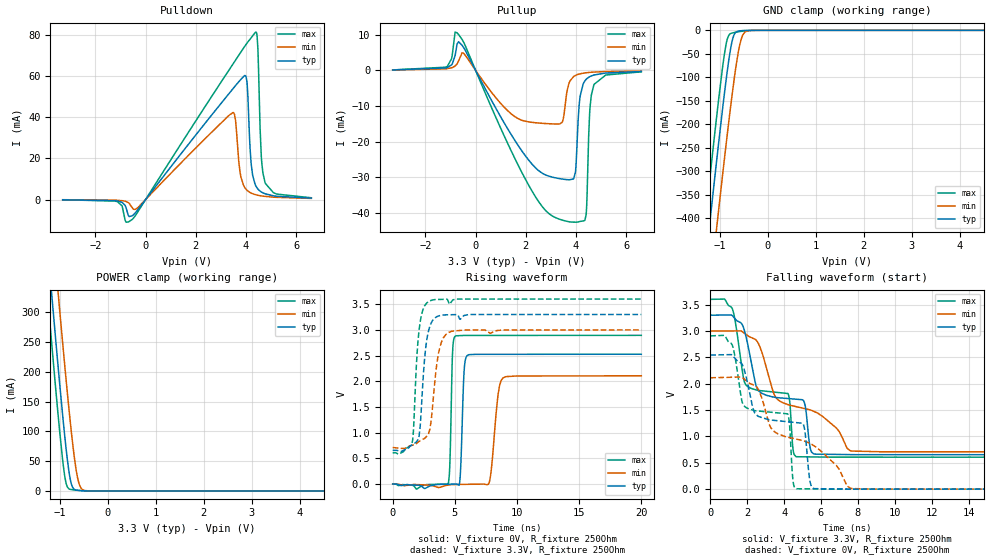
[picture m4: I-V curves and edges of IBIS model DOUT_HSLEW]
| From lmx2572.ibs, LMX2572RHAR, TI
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|   Model DOUT_HSLEW
[Model]   DOUT_HSLEW
Model_type   3-state
Polarity   Non-Inverting
Vmeas = 1.65
Vref = 3.3
Cref = 1pF
Rref = 250
|   typ   min   max
|   (nom PVT)   (fast PVT)   (slow PVT)
C_comp   1.019p   0.968p   1.051p
| Where nom  PVT is Nominal Process, 3.3V, 27C
|   Fast PVT is Strong Process,  3.6V, -40C
|   Slow PVT is Weak Process,   3V, 125C
[Voltage Range]   3.3   3   3.6
|Junction Temperature
[Temperature Range]   27   125   -40
[Pullup Reference]   3.3   3   3.6
[Pulldown Reference]   -0   0   -0
[Power Clamp Reference]   3.3   3   3.6
[GND Clamp Reference]   0   0   0
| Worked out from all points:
|   slope of the pulldown table from 0 to 0.495 V, typ, clamps not added: 63 ohm
|   slope of the pullup table from 0 to 0.495 V, typ, clamps not added: 74.7 ohm
|   GND clamp passes 1 mA (typ) near -0.57 V on its own axis
|   POWER clamp passes 1 mA (typ) near -0.63 V on its own axis
|   falling waveform, V_fixture 3.3V, R_fixture 250Ohm: 20-80 % time 3.26ns typ, 3.97ns min, 2.96ns max; typ from 3.3 V to 0.654 V
|   rising waveform, V_fixture 0V, R_fixture 250Ohm: 20-80 % time 206ps typ, 459ps min, 158ps max; typ from 0 V to 2.53 V
|   rising waveform, V_fixture 3.3V, R_fixture 250Ohm: 20-80 % time 493ps typ, 630ps min, 422ps max; typ from 0.657 V to 3.3 V
|   falling waveform, V_fixture 0V, R_fixture 250Ohm: 20-80 % time 3.28ns typ, 4.07ns min, 2.97ns max; typ from 2.54 V to 0 V
[Pulldown]
|   Voltage   I(typ)   I(min)   I(max)
-3.3V     -97.31uA   -66.38uA   -103.1uA
-537.9mV  -7.903mA   -3.884mA   -9.711mA
3.482V    53.83mA    42.24mA    65.82mA
3.759V    57.85mA    13.57mA    70.91mA
3.957V    60.23mA    5.716mA    74.52mA
4.046V    56.01mA    4.447mA    76.07mA
4.204V    17.43mA    3.161mA    78.53mA
4.392V    6.6mA      2.34mA     81.3mA
4.471V    5.142mA    2.107mA    73.28mA
4.61V     3.684mA    1.794mA    20.61mA
4.759V    2.815mA    1.546mA    8.205mA
6.6V      703.7uA    565.4uA    872.6uA
[GND Clamp]
|   Voltage   I(typ)   I(min)   I(max)
-3.3V     -2.452A    -2.589A    -2.364A
-1.439V   -627.2mA   -770.9mA   -533mA
-1.27V    -466.7mA   -610.7mA   -372.2mA
-1.211V   -410.7mA   -554.6mA   -316.2mA
-1.073V   -282mA     -425.3mA   -188.4mA
-1.033V   -246mA     -388.8mA   -153.2mA
-874.5mV  -109.2mA   -246.3mA   -31.62mA
-765.6mV  -33.07mA   -153.9mA   -6.398mA
-696.3mV  -7.92mA    -99.78mA   -4.642mA
-577.5mV  -1.073mA   -27.36mA   -2.516mA
-419.1mV  -88.15uA   -1.084mA   -769.1uA
6.6V      0A         0A         0A
[Pullup]
|   Voltage   I(typ)   I(min)   I(max)
-3.3V     103.2uA    82.1uA     106.6uA
-1.132V   773.6uA    462.9uA    1.092mA
-735.9mV  7.422mA    1.805mA    10.54mA
2.452V    -27.83mA   -14.78mA   -36.26mA
3.442V    -30.54mA   -14.66mA   -42.06mA
3.719V    -30.74mA   -3.65mA    -42.54mA
4.006V    -25.89mA   -1.343mA   -42.67mA
4.155V    -7.744mA   -993.3uA   -42.46mA
4.402V    -2.541mA   -687.5uA   -40.52mA
4.541V    -1.805mA   -585.3uA   -12.25mA
4.719V    -1.308mA   -490.8uA   -3.945mA
6.6V      -327.2uA   -179.6uA   -424.3uA
[POWER Clamp]
|   Voltage   I(typ)   I(min)   I(max)
-3.3V     2.408A     2.526A     2.331A
-1.389V   536.7mA    662mA      454.1mA
-1.231V   386.9mA    512.5mA    303.9mA
-1.171V   331.5mA    457.1mA    248.6mA
-1.053V   223.1mA    347.7mA    141.4mA
-1.013V   188mA      311.9mA    107.5mA
-894.3mV  88.96mA    207.3mA    22.7mA
-795.3mV  24.72mA    125.6mA    2.896mA
-735.9mV  6.329mA    81.34mA    1.968mA
-636.9mV  1.065mA    24.47mA    1.107mA
-478.5mV  181.4uA    709.5uA    176.1uA
6.6V      0A         0A         0A
[Ramp]
R_load = 250
|   typ   min   max
dV/dt_r   1.51618/2.06185e-10   1.26405/4.58899e-10   1.73655/1.57782e-10
dV/dt_f   1.58787/3.26139e-09   1.37589/3.97049e-09   1.79585/2.95886e-09
[Falling Waveform]
V_fixture = 3.3V
V_fixture_min = 3V
V_fixture_max = 3.6V
R_fixture = 250Ohm
C_fixture = 0F
|   Time   V(typ)   V(min)   V(max)
0s        3.3V       3V         3.6V
1.185ns   3.294V     3.001V     3.431V
1.908ns   2.931V     2.943V     1.99V
2.549ns   1.9V       2.799V     1.876V
4.216ns   1.719V     1.603V     1.814V
4.638ns   1.707V     1.567V     619mV
5.103ns   1.638V     1.529V     613.4mV
5.646ns   664.9mV    1.47V      611mV
7.635ns   655.2mV    723.3mV    607.1mV
20ns      653.6mV    706.9mV    606.9mV
[Rising Waveform]
V_fixture = 0V
V_fixture_min = 0V
V_fixture_max = 0V
R_fixture = 250Ohm
C_fixture = 0F
|   Time   V(typ)   V(min)   V(max)
0s        15.55nV    -303.8nV   26.96nV
4.451ns   -2.775mV   -19.97mV   -9.847mV
4.803ns   -1.285mV   -8.54mV    2.496V
5.03ns    -326.5uV   -7.751mV   2.877V
5.391ns   39.94mV    -6.492mV   2.889V
5.732ns   2.159V     -5.305mV   2.892V
6.045ns   2.51V      -4.216mV   2.892V
7.784ns   2.525V     48.56mV    2.893V
8.866ns   2.525V     2.063V     2.893V
20ns      2.527V     2.107V     2.894V
[Rising Waveform]
V_fixture = 3.3V
V_fixture_min = 3V
V_fixture_max = 3.6V
R_fixture = 250Ohm
C_fixture = 0F
|   Time   V(typ)   V(min)   V(max)
0s        656.7mV    711.1mV    609.3mV
1.559ns   764.3mV    754.9mV    804.1mV
1.665ns   780.4mV    762.9mV    1.022V
2.04ns    867.8mV    816.4mV    2.794V
2.208ns   1.114V     842.3mV    3.154V
2.628ns   2.594V     900.7mV    3.488V
2.926ns   3.021V     1.016V     3.559V
3.68ns    3.269V     2.539V     3.592V
4.483ns   3.294V     2.948V     3.547V
20ns      3.3V       3V         3.6V
[Falling Waveform]
|Gnd
V_fixture = 0V
V_fixture_min = 0V
V_fixture_max = 0V
R_fixture = 250Ohm
C_fixture = 0F
|   Time   V(typ)   V(min)   V(max)
0s        2.543V     2.112V     2.907V
1.185ns   2.542V     2.123V     2.739V
1.856ns   2.245V     2.084V     1.571V
2.411ns   1.443V     1.966V     1.49V
4.195ns   1.279V     986.7mV    1.429V
4.638ns   1.263V     951.7mV    11.81mV
5.073ns   1.202V     915.5mV    6.309mV
5.646ns   9.5mV      817mV      3.978mV
7.635ns   1.017mV    12.52mV    343.9uV
20ns      -36.48uV   -53.2uV    -27.43uV
